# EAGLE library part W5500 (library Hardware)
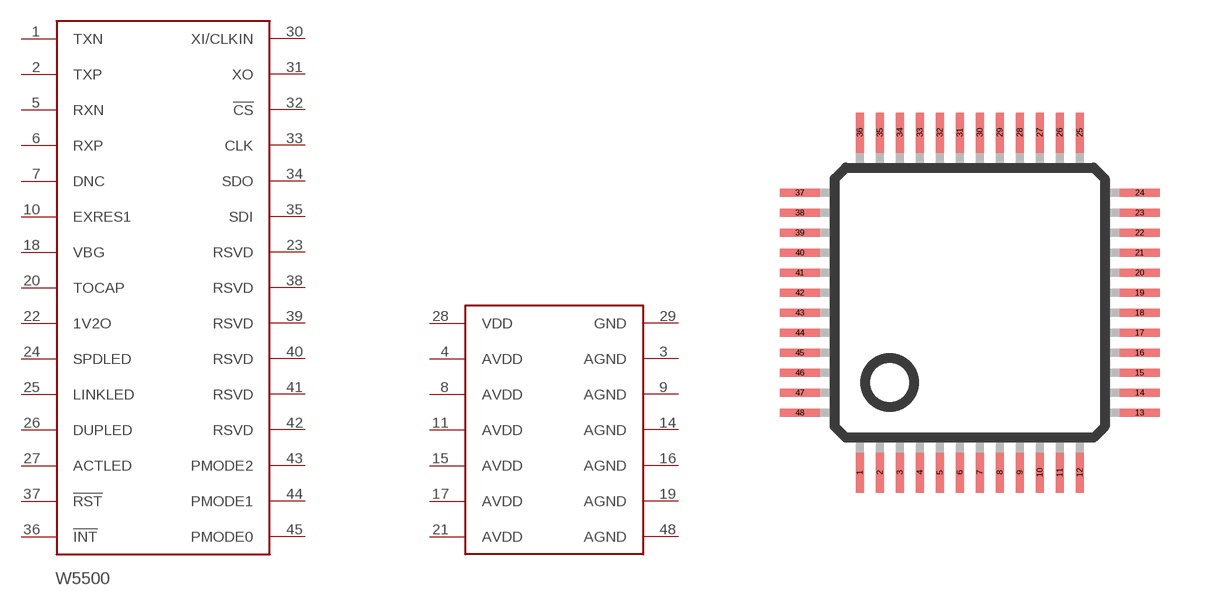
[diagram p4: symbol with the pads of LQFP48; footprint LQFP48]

Designator prefix -; gates G$1=W5500 G$2=W5500_PWR

## W5500  [LQFP48]
1  G$1:TXN
2  G$1:TXP
3  G$2:AGND
4  G$2:AVDD
5  G$1:RXN
6  G$1:RXP
7  G$1:DNC
8  G$2:AVDD
9  G$2:AGND
10  G$1:EXRES1
11  G$2:AVDD
14  G$2:AGND
15  G$2:AVDD
16  G$2:AGND
17  G$2:AVDD
18  G$1:VBG
19  G$2:AGND
20  G$1:TOCAP
21  G$2:AVDD
22  G$1:1V2O
23  G$1:RSVD
24  G$1:SPDLED
25  G$1:LINKLED
26  G$1:DUPLED
27  G$1:ACTLED
28  G$2:VDD
29  G$2:GND
30  G$1:XI/CLKIN
31  G$1:XO
32  G$1:!CS
33  G$1:CLK
34  G$1:SDO
35  G$1:SDI
36  G$1:!INT
37  G$1:!RST
38  G$1:RSVD
39  G$1:RSVD
40  G$1:RSVD
41  G$1:RSVD
42  G$1:RSVD
43  G$1:PMODE2
44  G$1:PMODE1
45  G$1:PMODE0
48  G$2:AGND

## Footprint LQFP48 (pad centres in mm)
48-pin plastic LQFP (FPT-48P-M26) www.fma.fujitsu.com/pdf/e713717.pdf
smd 0.2 x 1: 1 -2.75,-4.25; 2 -2.25,-4.25; 3 -1.75,-4.25; 4 -1.25,-4.25; 5 -0.75,-4.25; 6 -0.25,-4.25; 7 0.25,-4.25; 8 0.75,-4.25; 9 1.25,-4.25; 10 1.75,-4.25; 11 2.25,-4.25; 12 2.75,-4.25; 25 2.75,4.25; 26 2.25,4.25; 27 1.75,4.25; 28 1.25,4.25; 29 0.75,4.25; 30 0.25,4.25; 31 -0.25,4.25; 32 -0.75,4.25; 33 -1.25,4.25; 34 -1.75,4.25; 35 -2.25,4.25; 36 -2.75,4.25
smd 1 x 0.2: 13 4.25,-2.75; 14 4.25,-2.25; 15 4.25,-1.75; 16 4.25,-1.25; 17 4.25,-0.75; 18 4.25,-0.25; 19 4.25,0.25; 20 4.25,0.75; 21 4.25,1.25; 22 4.25,1.75; 23 4.25,2.25; 24 4.25,2.75; 37 -4.25,2.75; 38 -4.25,2.25; 39 -4.25,1.75; 40 -4.25,1.25; 41 -4.25,0.75; 42 -4.25,0.25; 43 -4.25,-0.25; 44 -4.25,-0.75; 45 -4.25,-1.25; 46 -4.25,-1.75; 47 -4.25,-2.25; 48 -4.25,-2.75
